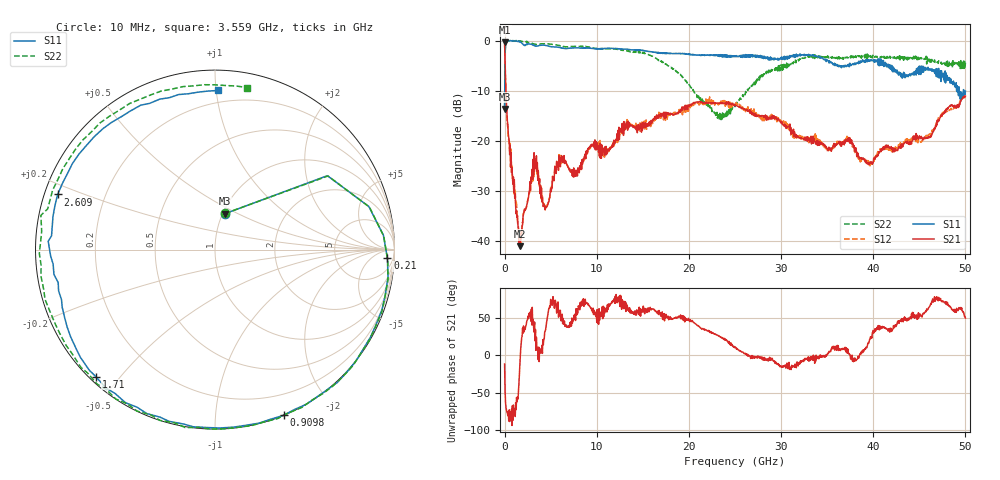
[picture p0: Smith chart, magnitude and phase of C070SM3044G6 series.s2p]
! 7/15/2021 9:15:19 AM
! Y:\C070SM3044G6\C070SM3044G6.S2P
! CHANNEL.1
! TR.MEASUREMENT
! CORRECTED.DATA
# GHZ S RI R 50.0
! FREQ.GHZ  S11RE  S11IM  S21RE  S21IM  S12RE  S12IM  S22RE  S22IM
!; PortSelection: Port_12
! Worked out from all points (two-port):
!   1001 points, 10 MHz to 50 GHz, reference 50 ohm
!   highest |S21| = -0.30 dB at 10 MHz (marker M1); lowest = -41.1 dB at 1.66 GHz (marker M2)
!   |S21| within 3 dB of the highest: start of sweep to 48.6 MHz
!   lowest |S11| = -13.7 dB at 10 MHz (marker M3), VSWR 1.52, Z = 51.3 + j21.5 ohm
!   |S11| at or under -10 dB: start of sweep to 26.38 MHz; 49.33 GHz to 49.79 GHz (464.4 MHz wide, 0.937 % of centre); 49.81034 GHz to end of sweep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
!   |S22| runs from -15.8 to 0.0 dB; largest |S21 - S12| = 0.038
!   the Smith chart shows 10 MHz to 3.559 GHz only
!   S11 on the Smith chart (normalised r, x): 10 MHz: 1.03, +0.43; 210 MHz: 20, -25; 909.8 MHz: 0.00, -1.50; 1.71 GHz: 0.02, -0.43; 2.609 GHz: 0.04, +0.17; 3.559 GHz: 0.12, +1.01
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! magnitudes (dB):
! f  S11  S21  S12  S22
! 10 MHz  -13.7  -0.3  -0.3  -13.6
! 210 MHz  -0.3  -12.7  -13.0  -0.3
! 909.8 MHz  0.0  -28.7  -27.5  0.0
! 1.66 GHz  -0.2  -41.1  -40.9  0.0
! 1.71 GHz  -0.3  -40.0  -40.4  -0.1
! 2.609 GHz  -0.6  -31.2  -31.1  -0.4
! 3.209 GHz  -1.0  -22.4  -23.0  -0.7
! 3.559 GHz  -1.0  -24.4  -25.1  -0.7
! 4.459 GHz  -0.9  -33.3  -33.1  -0.6
! 5.909 GHz  -1.3  -23.0  -22.8  -0.9
! 8.358 GHz  -1.5  -25.8  -25.4  -1.2
! 9.458 GHz  -1.5  -20.8  -20.7  -1.4
! 16.71 GHz  -2.3  -15.5  -15.3  -3.9
! 23.16 GHz  -2.9  -12.5  -12.6  -14.8
! 25 GHz  -3.2  -13.0  -12.6  -13.2
! 28.25 GHz  -3.2  -15.4  -16.0  -6.5
! 33.35 GHz  -3.0  -19.2  -19.3  -3.3
! 37.4 GHz  -5.2  -19.8  -19.4  -3.4
! 39.65 GHz  -4.1  -24.6  -25.0  -3.0
! 41.7 GHz  -4.8  -21.2  -21.9  -3.3
! 46.1 GHz  -5.6  -19.2  -18.7  -4.2
! 50 GHz  -10.0  -11.1  -11.3  -4.4
